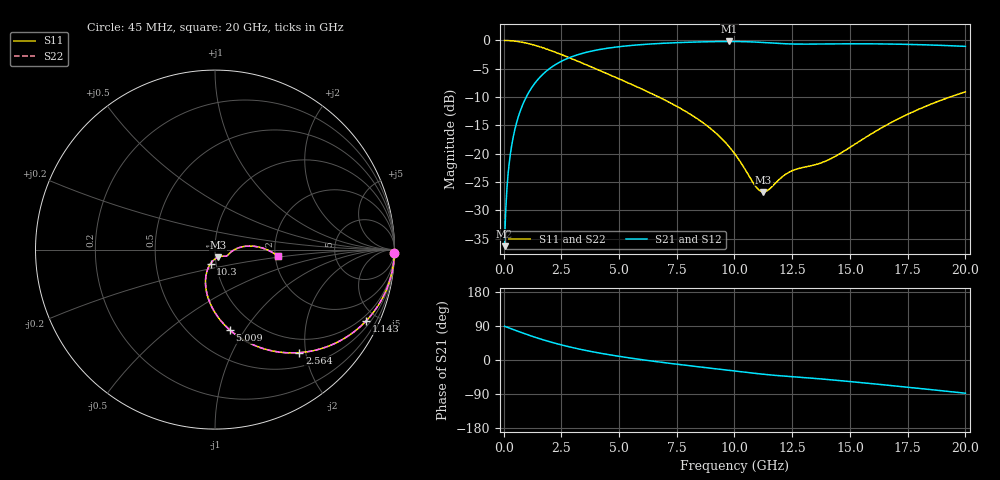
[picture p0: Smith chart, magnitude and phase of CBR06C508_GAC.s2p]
! S-parameter model data by Modelithics Inc.  support@modelithics.com 813-866-6335  Tampa FL USA
! S-Parameter data specifications:
! Substrate: 20-mil Rogers 4350B, substrate thickness, H=0.508mm, Dielectric constant, Er=3.75
! PCB Mounting Pad Footprint: Pad width, PadW=0.85mm , Pad length, PadL=0.64mm , Pad gap, PadG (edge-to-edge)=0.62mm , Reference planes=1.9mm apart
#  GHz  S  MA  R 50
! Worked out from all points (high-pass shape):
!   801 points, 45 MHz to 20 GHz, reference 50 ohm
!   highest |S21| = -0.18 dB at 9.773 GHz (marker M1); lowest = -36.3 dB at 45 MHz (marker M2)
!   |S21| within 3 dB of the highest: 2.767 GHz to end of sweep
!   lowest |S11| = -26.8 dB at 11.24 GHz (marker M3), VSWR 1.10, Z = 51.6 - j4.39 ohm
!   |S11| at or under -10 dB: 6.723 GHz to 19.33 GHz (12.6 GHz wide, 96.8 % of centre)
!   |S22| runs from -26.8 to 0.0 dB; largest |S21 - S12| = 0
!   S11 on the Smith chart (normalised r, x): 45 MHz: open; 1.143 GHz: 0.73, -4.35; 2.564 GHz: 0.74, -1.88; 5.009 GHz: 0.76, -0.86; 10.3 GHz: 0.94, -0.15; 20 GHz: 2.07, -0.17
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0.045  0.9999 -1.0  0.01523 89.0  0.01523 89.0  0.9999 -1.0
0.219606  0.9972 -5.0  0.07413 84.9  0.07413 84.9  0.9972 -5.0
0.294438  0.995 -6.7  0.09918 83.2  0.09918 83.2  0.995 -6.7
0.394213  0.9911 -9.0  0.1323 81.0  0.1323 81.0  0.9911 -9.0
0.693538  0.973 -15.7  0.2289 74.2  0.2289 74.2  0.973 -15.7
1.142525  0.931 -25.3  0.3621 64.6  0.3621 64.6  0.931 -25.3
1.816006  0.8465 -38.3  0.5279 51.4  0.5279 51.4  0.8465 -38.3
2.564319  0.7425 -50.7  0.6639 38.9  0.6639 38.9  0.7425 -50.7
3.387462  0.6337 -62.0  0.7666 27.4  0.7666 27.4  0.6337 -62.0
5.008806  0.4571 -79.4  0.8811 9.6  0.8811 9.6  0.4571 -79.4
6.704981  0.3175 -93.4  0.9394 -5.0  0.9394 -5.0  0.3175 -93.4
8.550819  0.1931 -105.9  0.9714 -18.7  0.9714 -18.7  0.1931 -105.9
9.773062  0.1148 -110.5  0.9791 -27.4  0.9791 -27.4  0.1148 -110.5
10.0225  0.09901 -109.9  0.9786 -29.2  0.9786 -29.2  0.09901 -109.9
10.29688  0.0821 -107.5  0.9769 -31.2  0.9769 -31.2  0.0821 -107.5
10.92047  0.05129 -88.2  0.9675 -35.5  0.9675 -35.5  0.05129 -88.2
11.24474  0.04589 -67.8  0.9595 -37.6  0.9595 -37.6  0.04589 -67.8
12.36721  0.06862 -32.1  0.932 -43.4  0.932 -43.4  0.06862 -32.1
13.36496  0.07861 -21.1  0.9286 -48.0  0.9286 -48.0  0.07861 -21.1
14.31283  0.09337 -6.4  0.9327 -53.0  0.9327 -53.0  0.09337 -6.4
16.68248  0.1834 6.1  0.93 -66.8  0.93 -66.8  0.1834 6.1
20  0.3519 -5.8  0.8865 -87.6  0.8865 -87.6  0.3519 -5.8
